|Texas Instruments Incorporated
|12/10/8-Bit, 1 MSPS, 16/12/8/4-Channel, Single-Ended, MicroPower,
|   Serial Interface ADCs
| Marketing part#   Voltage Range   Package-type   #pins
|ADS7950SDBT   1.7V - 5.25V   TSSOP   30-pin
|ADS7950SRGE   1.7V - 5.25V   QFN   24-pin
|ADS7951SDBT   1.7V - 5.25V   TSSOP   30-pin
|ADS7951SRGE   1.7V - 5.25V   QFN   24-pin
|ADS7952SDBT   1.7V - 5.25V   TSSOP   38-pin
|ADS7952SRHB   1.7V - 5.25V   QFN   32-pin
|ADS7953SDBT   1.7V - 5.25V   TSSOP   38-pin
|ADS7953SRHB   1.7V - 5.25V   QFN   32-pin
|ADS7954SDBT   1.7V - 5.25V   TSSOP   30-pin
|ADS7954SRGE   1.7V - 5.25V   QFN   24-pin
|ADS7955SDBT   1.7V - 5.25V   TSSOP   30-pin
|ADS7955SRGE   1.7V - 5.25V   QFN   30-pin
|ADS7956SDBT   1.7V - 5.25V   TSSOP   38-pin
|ADS7956SRHB   1.7V - 5.25V   QFN   24-pin
|ADS7957SDBT   1.7V - 5.25V   TSSOP   38-pin
|ADS7957SRHB   1.7V - 5.25V   QFN   32-pin
|ADS7958SDBT   1.7V - 5.25V   TSSOP   30-pin
|ADS7958SRGE   1.7V - 5.25V   QFN   24-pin
|ADS7959SDBT   1.7V - 5.25V   TSSOP   30-pin
|ADS7959SRGE   1.7V - 5.25V   QFN   24-pin
|ADS7960SDBT   1.7V - 5.25V   TSSOP   38-pin
|ADS7960SRHB   1.7V - 5.25V   QFN   32-pin
|ADS7961SDBT   1.7V - 5.25V   TSSOP   38-pin
|ADS7961SRHB   1.7V - 5.25V   QFN   32-pin
[IBIS Ver]   4.0
[File name]   ads795x.ibs
[File Rev]   1.0
[Date]   02/05/2010
[Source]   Texas Instruments Incorporated.
   Analog-eLab, HPA
   12500 TI Blvd
   Dallas, TX -75243
   For Support e-mail: elab_ibis@list.ti.com
[Notes]   Revision History:
   1.0: 02/05/2010
   - Initial version of the model
   - Initial Model generated from simulations in TISPICED
   - Model not matched to measurements
   - Ignore warnings related to ccomp, these are
   based on PVT variations as seen in simulations
   - The non-monotonic behavior with combined pulldown
   and pullp models for GPIO_3 and SDO_3 is inherent
   to buffers as seen in simulations.
[Disclaimer]
 This product is designed as an aid for customers of Texas Instruments.
 No warranties, either expressed or implied, with respect to this third
 party software (if any) or with respect to its fitness for any
 particular purpose is claimed by Texas Instruments or the author. The
 software (if any) is provided solely on an "as is" basis. The entire
 risk as to its quality and performance is with the customer
[Copyright] (C) Copyright 2009 Texas Instruments Incorporated.
   All rights reserved.
|   ADS7950, ADS7954, ADS7958
[Component]   ads7950_4_8sdbt   |30-pin TSSOP package
[Manufacturer] TI
[Package]
| variable   typ   min   max
R_pkg  0.083250   0.007080   0.123220
L_pkg  2.851241nH  1.247620nH  4.512760nH
C_pkg  0.317321pF  0.161550pF  0.549300pF
[Pin] signal_name  model_name  R_pin  L_pin C_pin
1   GPIO2  GPIO   0.12115  4.48656nH  0.54767pF
2   GPIO3  GPIO   0.12091  3.89544nH  0.44308pF
3   REFM   TERM   0.12104  3.27193nH  0.30290pF
4   REFP   TERM   0.11397  3.04645nH  0.28125pF
5   VA   TERM   0.04042  2.42961nH  0.35388pF
6   AGND   TERM   0.10289  2.82721nH  0.27532pF
7   MXO   TERM   0.09640  2.70201nH  0.26840pF
8   AINP   TERM   0.09512  2.67852nH  0.26714pF
9   AINM   TERM   0.09953  2.76540nH  0.27245pF
10  AGND   TERM   0.10878  2.94671nH  0.27434pF
11  NC   NC   0.00708  1.24762nH  0.16638pF
12  Ch3   TERM   0.10917  2.95772nH  0.25859pF
13  NC   NC   0.00721  1.33779nH  0.18180pF
14  Ch2   TERM   0.12322  3.94726nH  0.42431pF
15  NC   NC   0.01388  2.67964nH  0.43251pF
16  NC   NC   0.01388  2.67964nH  0.43251pF
17  NC   NC   0.01090  2.03716nH  0.31888pF
18  Ch1   TERM   0.11769  3.21119nH  0.28560pF
19  NC   NC   0.00708  1.25002nH  0.16155pF
20  Ch0   TERM   0.10389  2.85162nH  0.26866pF
21  VA   TERM   0.09695  2.71501nH  0.26668pF
22  AGND   TERM   0.09492  2.67430nH  0.25854pF
23  _CS   CS   0.09602  2.69622nH  0.26106pF
24  SCLK   SCLK   0.09531  2.68151nH  0.26682pF
25  SDI   SDI   0.10023  2.77571nH  0.27373pF
26  SDO   SDO   0.10989  2.96387nH  0.28266pF
27  BDGND  GND   0.06025  2.56699nH  0.33136pF
28  VBD   POWER   0.06402  2.76042nH  0.36506pF
29  GPIO0  GPIO   0.12322  3.94094nH  0.44720pF
30  GPIO1  GPIO   0.12248  4.51276nH  0.54930pF
[Component]   ads7950_4_8srge   |24-pin QFN package
[Manufacturer] TI
[Package]
| variable   typ   min   max
R_pkg  0.062430   0.000590   0.107430
L_pkg  1.154661nH   0.143390nH  1.917590nH
C_pkg  0.160173pF   0.077580pF  0.229250pF
[Pin] signal_name  model_name  R_pin  L_pin C_pin
1   VA   TERM   0.02899  1.07642nH  0.22925pF
2   AGND   TERM   0.08227  1.44643nH  0.18048pF
3   MXO   TERM   0.07836  1.37312nH  0.17661pF
4   AINP   TERM   0.08112  1.42432nH  0.18032pF
5   AINM   TERM   0.08992  1.58923nH  0.18403pF
6   NC   NC   0.00059  0.14339nH  0.07758pF
7   NC   NC   0.00059  0.14339nH  0.07759pF
8   Ch3   TERM   0.05974  1.03128nH  0.14705pF
9   Ch2   TERM   0.05567  0.95800nH  0.14317pF
10  Ch1   TERM   0.05535  0.95307nH  0.14372pF
11  Ch0   TERM   0.07817  1.36393nH  0.16941pF
12  NC   NC   0.00059  0.14339nH  0.07758pF
13  NC   NC   0.00059  0.14339nH  0.07759pF
14  VA   TERM   0.09747  1.72283nH  0.19123pF
15  AGND   TERM   0.09865  1.74452nH  0.19167pF
16  _CS   CS   0.09733  1.71941nH  0.19217pF
17  SCLK   SCLK   0.09997  1.77023nH  0.20186pF
18  SDI   SDI   0.10743  1.91759nH  0.19550pF
19  SDO   SDO   0.10091  1.79529nH  0.18618pF
20  BDGND  GND   0.07593  1.32243nH  0.17386pF
21  VDB   POWER   0.01951  0.64435nH  0.19739pF
22  GPIO   GPIO   0.05678  0.97914nH  0.14755pF
23  REFM   TERM   0.05694  0.98274nH  0.14597pF
24  REFP   TERM   0.07544  1.32398nH  0.15638pF
|   ADS7951, ADS7955, and ADS7959
[Component]   ads7951_5_9sdbt   |30-pin TSSOP package
[Manufacturer] TI
[Package]
| variable   typ   min   max
R_pkg  0.083250   0.007080   0.123220
L_pkg  2.851241nH  1.247620nH  4.512760nH
C_pkg  0.317321pF  0.161550pF  0.549300pF
[Pin] signal_name  model_name  R_pin  L_pin C_pin
1   GPIO2  GPIO   0.12115  4.48656nH  0.54767pF
2   GPIO3  GPIO   0.12091  3.89544nH  0.44308pF
3   REFM   TERM   0.12104  3.27193nH  0.30290pF
4   REFP   TERM   0.11397  3.04645nH  0.28125pF
5   VA   TERM   0.04042  2.42961nH  0.35388pF
6   AGND   TERM   0.10289  2.82721nH  0.27532pF
7   MXO   TERM   0.09640  2.70201nH  0.26840pF
8   AINP   TERM   0.09512  2.67852nH  0.26714pF
9   AINM   TERM   0.09953  2.76540nH  0.27245pF
10  AGND   TERM   0.10878  2.94671nH  0.27434pF
11  Ch7   TERM   0.00708  1.24762nH  0.16638pF
12  Ch6   TERM   0.10917  2.95772nH  0.25859pF
13  Ch5   TERM   0.00721  1.33779nH  0.18180pF
14  Ch4   TERM   0.12322  3.94726nH  0.42431pF
15  NC   NC   0.01388  2.67964nH  0.43251pF
16  NC   NC   0.01388  2.67964nH  0.43251pF
17  Ch3   TERM   0.01090  2.03716nH  0.31888pF
18  Ch2   TERM   0.11769  3.21119nH  0.28560pF
19  Ch1   TERM   0.00708  1.25002nH  0.16155pF
20  Ch0   TERM   0.10389  2.85162nH  0.26866pF
21  VA   TERM   0.09695  2.71501nH  0.26668pF
22  AGND   TERM   0.09492  2.67430nH  0.25854pF
23  _CS   CS   0.09602  2.69622nH  0.26106pF
24  SCLK   SCLK   0.09531  2.68151nH  0.26682pF
25  SDI   SDI   0.10023  2.77571nH  0.27373pF
26  SDO   SDO   0.10989  2.96387nH  0.28266pF
27  BDGND  GND   0.06025  2.56699nH  0.33136pF
28  VBD   POWER   0.06402  2.76042nH  0.36506pF
29  GPIO0  GPIO   0.12322  3.94094nH  0.44720pF
30  GPIO1  GPIO   0.12248  4.51276nH  0.54930pF
[Component]   ads7951_5_9srge   |24-pin QFN package
[Manufacturer] TI
[Package]
| variable   typ   min   max
R_pkg  0.062430   0.000590   0.107430
L_pkg  1.154661nH   0.143390nH  1.917590nH
C_pkg  0.160173pF   0.077580pF  0.229250pF
[Pin] signal_name  model_name  R_pin  L_pin C_pin
1   VA   TERM   0.02899  1.07642nH  0.22925pF
2   AGND   TERM   0.08227  1.44643nH  0.18048pF
3   MXO   TERM   0.07836  1.37312nH  0.17661pF
4   AINP   TERM   0.08112  1.42432nH  0.18032pF
5   AINM   TERM   0.08992  1.58923nH  0.18403pF
6   Ch7   TERM   0.00059  0.14339nH  0.07758pF
7   Ch6   TERM   0.00059  0.14339nH  0.07759pF
8   Ch5   TERM   0.05974  1.03128nH  0.14705pF
9   Ch4   TERM   0.05567  0.95800nH  0.14317pF
10  Ch3   TERM   0.05535  0.95307nH  0.14372pF
11  Ch2   TERM   0.07817  1.36393nH  0.16941pF
12  Ch1   TERM   0.00059  0.14339nH  0.07758pF
13  Ch0   TERM   0.00059  0.14339nH  0.07759pF
14  VA   TERM   0.09747  1.72283nH  0.19123pF
15  AGND   TERM   0.09865  1.74452nH  0.19167pF
16  _CS   CS   0.09733  1.71941nH  0.19217pF
17  SCLK   SCLK   0.09997  1.77023nH  0.20186pF
18  SDI   SDI   0.10743  1.91759nH  0.19550pF
19  SDO   SDO   0.10091  1.79529nH  0.18618pF
20  BDGND  GND   0.07593  1.32243nH  0.17386pF
21  VDB   POWER   0.01951  0.64435nH  0.19739pF
22  GPIO   GPIO   0.05678  0.97914nH  0.14755pF
23  REFM   TERM   0.05694  0.98274nH  0.14597pF
24  REFP   TERM   0.07544  1.32398nH  0.15638pF
|   ADS7952, ADS7956, and ADS7960
[Component]   ads7952_56_60sdbt   |38-pin TSSOP package
[Manufacturer] TI
[Package]
| variable   typ   min   max
R_pkg  0.110493   0.007830   0.163170
L_pkg  3.320391nH   1.142020nH   5.189470nH
C_pkg  0.564484pF   0.356000pF   0.797790pF
[Pin] signal_name  model_name  R_pin  L_pin C_pin
1   GPIO2   GPIO   0.13142  4.54931nH  0.70932pF
2   GPIO3   GPIO   0.12989  4.23911nH  0.75619pF
3   REFM   TERM   0.12955  3.96838nH  0.69068pF
4   REFP   TERM   0.14132  3.78231nH  0.57054pF
5   VA   TERM   0.07003  2.78305nH  0.55809pF
6   AGND   TERM   0.06536  2.58840nH  0.56557pF
7   MXO   TERM   0.11384  2.92151nH  0.48279pF
8   AINP   TERM   0.10407  2.73102nH  0.46734pF
9   AINM   TERM   0.09885  2.63089nH  0.45949pF
10  AGND   TERM   0.09903  2.63561nH  0.45183pF
11  NC   NC   0.00784  1.14231nH  0.35601pF
12  NC   NC   0.00783  1.14202nH  0.35610pF
13  NC   NC   0.00784  1.14263nH  0.35600pF
14  NC   NC   0.00783  1.14285nH  0.35602pF
15  Ch11   TERM   0.13747  3.39683nH  0.47885pF
16  Ch10   TERM   0.15944  4.15234nH  0.59561pF
17  Ch9   TERM   0.16028  4.58758nH  0.73330pF
18  Ch8   TERM   0.16138  4.87886nH  0.79760pF
19  AGND   TERM   0.16317  5.18947nH  0.74710pF
20  AGND   TERM   0.16317  5.18947nH  0.74716pF
21  Ch7   TERM   0.16138  4.87886nH  0.79779pF
22  Ch6   TERM   0.16028  4.58758nH  0.73378pF
23  Ch5   TERM   0.15944  4.15234nH  0.59728pF
24  Ch4   TERM   0.13747  3.39683nH  0.49550pF
25  Ch3   TERM   0.12133  3.07505nH  0.49150pF
26  Ch2   TERM   0.10945  2.84073nH  0.47524pF
27  Ch1   TERM   0.10135  2.68142nH  0.46392pF
28  Ch0   TERM   0.09825  2.62001nH  0.45872pF
29  VA   TERM   0.10047  2.66161nH  0.46001pF
30  AGND   TERM   0.10715  2.79089nH  0.46059pF
31  _CS   CS   0.10170  2.68542nH  0.45710pF
32  SCLK   SCLK   0.11006  2.84771nH  0.47499pF
33  SDI   SDI   0.12212  3.08414nH  0.49161pF
34  SDO   SDO   0.13840  3.40726nH  0.49420pF
35  BDGND   GND   0.07509  3.31165nH  0.63430pF
36  VBD   POWER   0.07127  3.51959nH  0.75886pF
37  GPIO0   GPIO   0.13151  4.27101nH  0.75883pF
38  GPIO1   GPIO   0.13241  4.56881nH  0.71058pF
[Component]   ads7952_56_60srhb   |32-pin QFN package
[Manufacturer] TI
[Package]
| variable   typ   min   max
R_pkg  0.085267   0.000190   0.149040
L_pkg  1.504003nH  0.054810nH  2.634060nH
C_pkg  0.146941pF  0.044080pF  0.218090pF
[Pin] signal_name  model_name  R_pin  L_pin C_pin
1   AGND   TERM   0.05493  1.40765nH  0.21809pF
2   MXO   TERM   0.09556  1.62060nH  0.15564pF
3   AINP   TERM   0.08636  1.44762nH  0.14034pF
4   AINM   TERM   0.08261  1.37781nH  0.12929pF
5   NC   NC   0.00019  0.05481nH  0.04408pF
6   NC   NC   0.00019  0.05491nH  0.04408pF
7   Ch11   TERM   0.08416  1.40710nH  0.13459pF
8   Ch10   TERM   0.10354  1.77445nH  0.15453pF
9   Ch9   TERM   0.10451  1.79206nH  0.15541pF
10  Ch8   TERM   0.08750  1.46770nH  0.14074pF
11  Ch7   TERM   0.08294  1.38131nH  0.13304pF
12  Ch6   TERM   0.07889  1.30431nH  0.13103pF
13  Ch5   TERM   0.08156  1.35231nH  0.13524pF
14  Ch4   TERM   0.09021  1.51312nH  0.14796pF
15  Ch3   TERM   0.10998  1.88619nH  0.17783pF
16  Ch2   TERM   0.13714  2.40646nH  0.19800pF
17  Ch1   TERM   0.14604  2.57636nH  0.20027pF
18  Ch0   TERM   0.13216  2.30770nH  0.18523pF
19  NC   NC   0.00019  0.05491nH  0.04408pF
20  NC   NC   0.00019  0.05481nH  0.04408pF
21  VA   TERM   0.13272  2.31781nH  0.18247pF
22  AGND   TERM   0.14025  2.46232nH  0.18953pF
23  _CS   CS   0.13429  2.34851nH  0.18730pF
24  SCLK   SCLK   0.14904  2.63406nH  0.20384pF
25  SDI   SDI   0.14115  2.48346nH  0.20167pF
26  SDO   SDO   0.11433  1.96910nH  0.17718pF
27  BDGND  GND   0.08786  1.46891nH  0.14184pF
28  VBD   POWER   0.02209  0.69397nH  0.16917pF
29  GPIO   GPIO   0.06117  0.97983nH  0.10668pF
30  REFM   TERM   0.06114  0.97943nH  0.10477pF
31  REFP   TERM   0.07543  1.24190nH  0.12786pF
32  VA   TERM   0.05022  1.30661nH  0.19626pF
|   ADS7953, ADS7957, ADS7961
[Component]   ads7953_57_61sdbt   |38-pin TSSOP package
[Manufacturer] TI
[Package]
| variable   typ   min   max
R_pkg  0.110493   0.007830   0.163170
L_pkg  3.320391nH   1.142020nH   5.189470nH
C_pkg  0.564484pF   0.356000pF   0.797790pF
[Pin] signal_name  model_name  R_pin  L_pin C_pin
1   GPIO2   GPIO   0.13142  4.54931nH  0.70932pF
2   GPIO3   GPIO   0.12989  4.23911nH  0.75619pF
3   REFM   TERM   0.12955  3.96838nH  0.69068pF
4   REFP   TERM   0.14132  3.78231nH  0.57054pF
5   VA   TERM   0.07003  2.78305nH  0.55809pF
6   AGND   TERM   0.06536  2.58840nH  0.56557pF
7   MXO   TERM   0.11384  2.92151nH  0.48279pF
8   AINP   TERM   0.10407  2.73102nH  0.46734pF
9   AINM   TERM   0.09885  2.63089nH  0.45949pF
10  AGND   TERM   0.09903  2.63561nH  0.45183pF
11  CH15   TERM   0.00784  1.14231nH  0.35601pF
12  CH14   TERM   0.00783  1.14202nH  0.35610pF
13  CH13   TERM   0.00784  1.14263nH  0.35600pF
14  CH12   TERM   0.00783  1.14285nH  0.35602pF
15  Ch11   TERM   0.13747  3.39683nH  0.47885pF
16  Ch10   TERM   0.15944  4.15234nH  0.59561pF
17  Ch9   TERM   0.16028  4.58758nH  0.73330pF
18  Ch8   TERM   0.16138  4.87886nH  0.79760pF
19  AGND   TERM   0.16317  5.18947nH  0.74710pF
20  AGND   TERM   0.16317  5.18947nH  0.74716pF
21  Ch7   TERM   0.16138  4.87886nH  0.79779pF
22  Ch6   TERM   0.16028  4.58758nH  0.73378pF
23  Ch5   TERM   0.15944  4.15234nH  0.59728pF
24  Ch4   TERM   0.13747  3.39683nH  0.49550pF
25  Ch3   TERM   0.12133  3.07505nH  0.49150pF
26  Ch2   TERM   0.10945  2.84073nH  0.47524pF
27  Ch1   TERM   0.10135  2.68142nH  0.46392pF
28  Ch0   TERM   0.09825  2.62001nH  0.45872pF
29  VA   TERM   0.10047  2.66161nH  0.46001pF
30  AGND   TERM   0.10715  2.79089nH  0.46059pF
31  _CS   CS   0.10170  2.68542nH  0.45710pF
32  SCLK   SCLK   0.11006  2.84771nH  0.47499pF
33  SDI   SDI   0.12212  3.08414nH  0.49161pF
34  SDO   SDO   0.13840  3.40726nH  0.49420pF
35  BDGND   GND   0.07509  3.31165nH  0.63430pF
36  VBD   POWER   0.07127  3.51959nH  0.75886pF
37  GPIO0   GPIO   0.13151  4.27101nH  0.75883pF
38  GPIO1   GPIO   0.13241  4.56881nH  0.71058pF|
[Component]   ads7953_57_61srhb   |32-pin QFN package
[Manufacturer] TI
[Package]
| variable   typ   min   max
R_pkg  0.085267   0.000190   0.149040
L_pkg  1.504003nH  0.054810nH  2.634060nH
C_pkg  0.146941pF  0.044080pF  0.218090pF
[Pin] signal_name  model_name  R_pin  L_pin C_pin
1   AGND   TERM   0.05493  1.40765nH  0.21809pF
2   MXO   TERM   0.09556  1.62060nH  0.15564pF
3   AINP   TERM   0.08636  1.44762nH  0.14034pF
4   AINM   TERM   0.08261  1.37781nH  0.12929pF
5   CH15   TERM   0.00019  0.05481nH  0.04408pF
6   CH14   TERM   0.00019  0.05491nH  0.04408pF
7   Ch13   TERM   0.08416  1.40710nH  0.13459pF
8   Ch12   TERM   0.10354  1.77445nH  0.15453pF
9   Ch11   TERM   0.10451  1.79206nH  0.15541pF
10  Ch10   TERM   0.08750  1.46770nH  0.14074pF
11  Ch9   TERM   0.08294  1.38131nH  0.13304pF
12  Ch8   TERM   0.07889  1.30431nH  0.13103pF
13  Ch7   TERM   0.08156  1.35231nH  0.13524pF
14  Ch6   TERM   0.09021  1.51312nH  0.14796pF
15  Ch5   TERM   0.10998  1.88619nH  0.17783pF
16  Ch4   TERM   0.13714  2.40646nH  0.19800pF
17  Ch3   TERM   0.14604  2.57636nH  0.20027pF
18  Ch2   TERM   0.13216  2.30770nH  0.18523pF
19  CH1   TERM   0.00019  0.05491nH  0.04408pF
20  CH0   TERM   0.00019  0.05481nH  0.04408pF
21  VA   TERM   0.13272  2.31781nH  0.18247pF
22  AGND   TERM   0.14025  2.46232nH  0.18953pF
23  _CS   CS   0.13429  2.34851nH  0.18730pF
24  SCLK   SCLK   0.14904  2.63406nH  0.20384pF
25  SDI   SDI   0.14115  2.48346nH  0.20167pF
26  SDO   SDO   0.11433  1.96910nH  0.17718pF
27  BDGND  GND   0.08786  1.46891nH  0.14184pF
28  VBD   POWER   0.02209  0.69397nH  0.16917pF
29  GPIO   GPIO   0.06117  0.97983nH  0.10668pF
30  REFM   TERM   0.06114  0.97943nH  0.10477pF
31  REFP   TERM   0.07543  1.24190nH  0.12786pF
32  VA   TERM   0.05022  1.30661nH  0.19626pF
|   Model Selectors
[Model Selector]  CS
CS_3   3.3V digital input
CS_5   5V digital input
[Model Selector]  SCLK
SCLK_3  3.3V digital input
SCLK_5  5V digital input
[Model Selector]  SDI
SDI_3   3.3V digital input
SDI_5   5V digital input
[Model Selector]  SDO
SDO_3   3.3V digital 3-state
SDO_5   5V digital 3-state
[Model Selector]  GPIO
GPIO_3   3.3V digital I/O
GPIO_5   5V digital I/O
|   TERM Model
[Model] TERM
Model_type Terminator
C_comp   0   0   0
| variable   typ   min   max
[Voltage Range]   3.3V   1.7V   5.25V
[POWER Clamp Reference]  3.3V   1.7V   5.25V
[GND Clamp Reference]   0.0V   0.0V   0.0V
|Operating Temperature
[Temperature Range]   27   85   -40
| Models and submodels in the file (11): TERM (Terminator), CS_3 (Input), CS_5 (Input), SCLK_3 (Input), SCLK_5 (Input), SDI_3 (Input), SDI_5 (Input), SDO_3 (3-state), SDO_5 (3-state), GPIO_3 (I/O), GPIO_5 (I/O)
